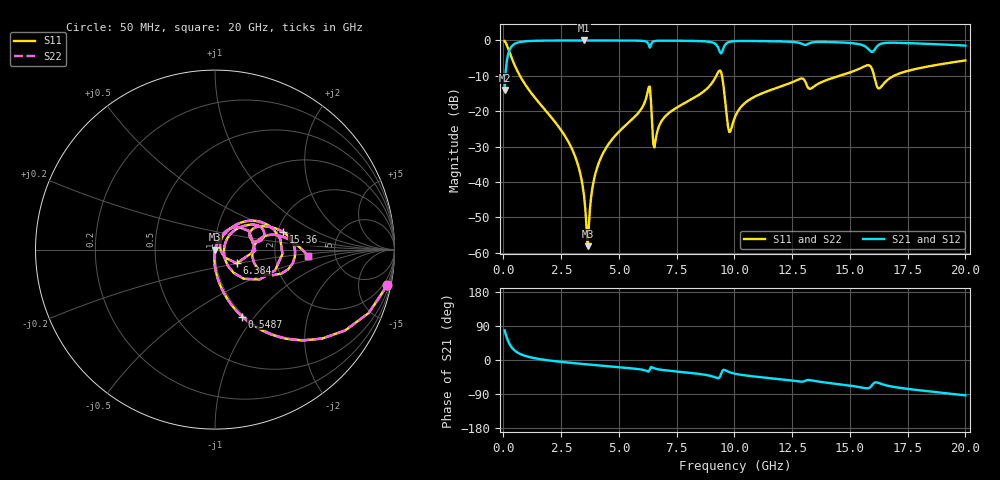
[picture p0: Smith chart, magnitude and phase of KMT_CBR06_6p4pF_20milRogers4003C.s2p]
! Data measured by Modelithics Inc. support@modelithics.com 813-866-6335
! KEMET CBR0603 6.4pF, Pad Width= 0.851mm, Pad Length= 0.64mm, Pad Gap= 0.62mm, 20mil Rogers 4003C substrate Data, January 2022
# hz S ma R 50
! 2 Port Network Data from SP1.SP block
! freq  magS11  angS11  magS21  angS21  magS12  angS12  magS22  angS22
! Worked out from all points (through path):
!   401 points, 50 MHz to 20 GHz, reference 50 ohm
!   highest |S21| = -0.01 dB at 3.491 GHz (marker M1); lowest = -14.0 dB at 50 MHz (marker M2)
!   group delay of S21, straight-line fit = 14.4 ps
!   lowest |S11| = -58.1 dB at 3.641 GHz (marker M3), VSWR 1.00, Z = 50.1 - j0.0342 ohm
!   |S11| at or under -10 dB: 712.4 MHz to 9.214 GHz (8.502 GHz wide, 171 % of centre); 9.46 GHz to 14.55 GHz (5.093 GHz wide, 42.4 % of centre); 16.05 GHz to 16.91 GHz (860.3 MHz wide, 5.22 % of centre)
!   |S22| runs from -58.1 to -0.2 dB; largest |S21 - S12| = 0
!   S11 on the Smith chart (normalised r, x): 50 MHz: 0.98, -9.72; 548.8 MHz: 0.97, -0.87; 6.384 GHz: 1.26, -0.20; 15.36 GHz: 2.14, +0.50; 20 GHz: 3.14, -0.33
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5e7  0.98 -11.6  0.1989 78.4  0.1989 78.4  0.98 -11.6
2.495e8  0.7008 -46.3  0.7128 43.7  0.7128 43.7  0.7008 -46.3
5.4875e8  0.4021 -68.0  0.915 21.9  0.915 21.9  0.4021 -68.0
2.74325e9  0.0403 -95.0  0.998 -6.5  0.998 -6.5  0.0403 -95.0
3.391625e9  0.01034 -93.7  0.9986 -10.3  0.9986 -10.3  0.01034 -93.7
3.491375e9  0.00625 -89.7  0.9987 -10.8  0.9987 -10.8  0.00625 -89.7
3.641e9  0.001238 -16.0  0.9986 -11.7  0.9986 -11.7  0.001238 -16.0
3.94025e9  0.0116 70.3  0.9985 -13.3  0.9985 -13.3  0.0116 70.3
4.33925e9  0.02646 71.6  0.9981 -15.4  0.9981 -15.4  0.02646 71.6
6.2345e9  0.182 43.8  0.9334 -30.0  0.9334 -30.0  0.182 43.8
6.384125e9  0.1431 -32.2  0.8602 -18.4  0.8602 -18.4  0.1431 -32.2
6.53375e9  0.03078 23.0  0.9778 -22.1  0.9778 -22.1  0.03078 23.0
6.73325e9  0.06117 58.0  0.9905 -24.9  0.9905 -24.9  0.06117 58.0
9.32675e9  0.3683 9.1  0.7487 -47.5  0.7487 -47.5  0.3683 9.1
9.775625e9  0.05064 -9.7  0.9526 -32.1  0.9526 -32.1  0.05064 -9.7
1.0025e10  0.08266 39.6  0.9764 -36.4  0.9764 -36.4  0.08266 39.6
1.137162e10  0.1884 41.5  0.9759 -46.8  0.9759 -46.8  0.1884 41.5
1.336662e10  0.2138 25.1  0.9374 -54.2  0.9374 -54.2  0.2138 25.1
1.536162e10  0.3919 14.5  0.8896 -71.1  0.8896 -71.1  0.3919 14.5
1.601e10  0.3508 -24.0  0.7013 -62.7  0.7013 -62.7  0.3508 -24.0
1.670825e10  0.2898 15.2  0.927 -68.9  0.927 -68.9  0.2898 15.2
2e10  0.5211 -4.2  0.8444 -93.3  0.8444 -93.3  0.5211 -4.2
